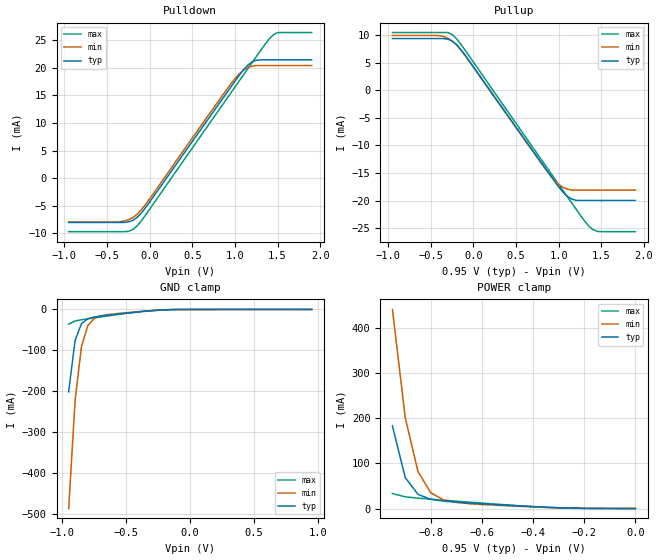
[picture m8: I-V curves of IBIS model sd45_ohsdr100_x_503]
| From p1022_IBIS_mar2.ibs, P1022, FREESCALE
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[Model]   sd45_ohsdr100_x_503
Model_type 3-state
Enable Active-High
Polarity Non-Inverting
|   TYP   MIN   MAX
C_comp   1.60pF   1.60pF   1.67pF
[Model Spec]
Vmeas   0.475   0.425   0.605
[Voltage Range]   0.95   0.85   1.21
[Temperature Range] 65   125   -40
[Driver Schedule]
| Model_Name  Rise_on_dly   Rise_off_dly   Fall_on_dly   Fall_off_dly
sd45_ohsdr100_x_50   0ps   NA   0ps   NA
sd45_ohsdr100_x_53  333.33ps   NA  333.33ps   NA
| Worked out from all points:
|   slope of the pulldown table from 0 to 0.142 V, typ, clamps not added: 45.7 ohm
|   slope of the pullup table from 0 to 0.142 V, typ, clamps not added: 45.5 ohm
|   GND clamp passes 1 mA (typ) near -0.19 V on its own axis
|   POWER clamp passes 1 mA (typ) near -0.25 V on its own axis
[Pullup]
|   Vout(V)   TYP   WCS   BCS
-950mV    9.394mA    9.972mA    10.49mA
-400mV    9.394mA    9.921mA    10.49mA
-250mV    8.951mA    8.974mA    10.15mA
-100mV    6.461mA    6.356mA    7.34mA
800mV     -13.2mA    -13.28mA   -12.64mA
1V        -17.5mA    -17.05mA   -17.05mA
1.1V      -19.21mA   -17.92mA   -19.26mA
1.15V     -19.7mA    -18.08mA   -20.36mA
1.3V      -19.98mA   -18.11mA   -23.62mA
1.4V      -19.98mA   -18.11mA   -25.24mA
1.5V      -19.98mA   -18.11mA   -25.64mA
1.9V      -19.98mA   -18.11mA   -25.64mA
[Pulldown]
|   Vout(V)   TYP   WCS   BCS
-950mV    -8.027mA   -7.945mA   -9.693mA
-350mV    -8.027mA   -7.908mA   -9.693mA
-250mV    -7.938mA   -7.555mA   -9.642mA
-150mV    -7.144mA   -6.573mA   -8.705mA
0V        -4.323mA   -3.744mA   -5.622mA
950mV     16.44mA    17.03mA    15.39mA
1.1V      19.6mA     19.57mA    18.69mA
1.2V      21.04mA    20.28mA    20.89mA
1.25V     21.36mA    20.39mA    21.99mA
1.45V     21.44mA    20.39mA    25.96mA
1.5V      21.44mA    20.39mA    26.36mA
1.9V      21.44mA    20.39mA    26.38mA
[GND Clamp]
|   Vout(V)   TYP   WCS   BCS
-950mV    -201.6mA   -486.5mA   -36.16mA
-900mV    -75.75mA   -222.9mA   -28.05mA
-850mV    -34.66mA   -90.59mA   -25.11mA
-800mV    -22.71mA   -39.37mA   -22.78mA
-750mV    -18.57mA   -21.91mA   -20.52mA
-700mV    -16.25mA   -15.71mA   -18.29mA
-650mV    -14.32mA   -12.88mA   -16.07mA
-400mV    -5.858mA   -5.175mA   -5.911mA
-200mV    -1.108mA   -1.072mA   -756.7uA
950mV     70.01uA    122.9uA    16.34uA
[POWER Clamp]
|   Vout(V)   TYP   WCS   BCS
-950mV    183.5mA    442.2mA    33.42mA
-900mV    68.86mA    202.2mA    25.88mA
-850mV    31.34mA    81.75mA    23.04mA
-800mV    20.35mA    35.06mA    20.76mA
-750mV    16.45mA    19.08mA    18.55mA
-700mV    14.21mA    13.35mA    16.36mA
-650mV    12.35mA    10.71mA    14.18mA
-300mV    1.805mA    1.559mA    1.409mA
0V        0A         0A         0A
[Ramp]
R_load=50.00
dV/dt_r  1.7449e-01/6.4215e-11  1.5361e-01/6.5528e-11  2.2871e-01/6.5586e-11
dV/dt_f  1.7449e-01/6.5823e-11  1.5361e-01/6.7896e-11  2.2872e-01/6.6497e-11
